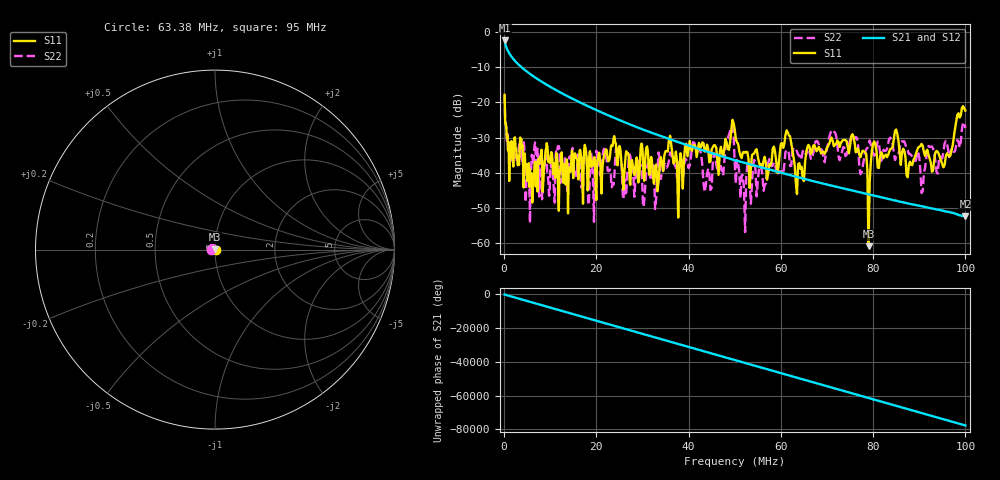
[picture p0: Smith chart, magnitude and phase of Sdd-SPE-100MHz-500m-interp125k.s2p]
!Keysight Technologies PLTS 2019, Build 20190114.1
!FILE: C:\Users\fxb06141\Documents\BUREAU - 2022\IEEE802.3\IEEE802.3dg\Cable modeling\125kHz Interpolation\SPE-100MHz-500m-interp125k.s4p
!$DUT_CFG_DESC: Default 4-Port Configuration
!$NUMBER_PORTS: 4
!$DIFF_PORT_MAP: 1|2P|2|2P|0|UC|0|UC|
!$PORT_MAP: 1|1|<<<<<<|2|2|>>>>>>|3|3|<<<<<<|4|4|>>>>>>|
!Date: Tuesday, March 05, 2024, 10:46:46
!S2P File: Measurements: SDD11,SDD12,SDD21,SDD22:
# MHz S  RI  R 50
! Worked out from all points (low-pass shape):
!   800 points, 125 kHz to 100 MHz, reference 50 ohm
!   highest |S21| = -2.50 dB at 125 kHz (marker M1); lowest = -52.3 dB at 100 MHz (marker M2)
!   |S21| within 3 dB of the highest: start of sweep to 858.2 kHz
!   lowest |S11| = -60.8 dB at 79 MHz (marker M3), VSWR 1.00, Z = 50 + j0.0913 ohm
!   |S11| at or under -10 dB: start of sweep to end of sweep
!   |S22| runs from -56.8 to -18.1 dB; largest |S21 - S12| = 0
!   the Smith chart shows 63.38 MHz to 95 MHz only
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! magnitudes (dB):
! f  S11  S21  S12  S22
! 125 kHz  -17.9  -2.5  -2.5  -18.1
! 1.5 MHz  -32.7  -6.9  -6.9  -31.2
! 5.125 MHz  -37.6  -11.5  -11.5  -40.4
! 6.375 MHz  -41.6  -12.7  -12.7  -37.5
! 16.88 MHz  -38.5  -20.3  -20.3  -43.7
! 23.75 MHz  -30.3  -24.4  -24.4  -43.3
! 33.5 MHz  -42.5  -29.4  -29.4  -34.2
! 41.5 MHz  -32.5  -32.9  -32.9  -32.3
! 43.62 MHz  -33.8  -33.9  -33.9  -44.5
! 49.25 MHz  -27.9  -36.2  -36.2  -27.1
! 50.12 MHz  -29.1  -36.5  -36.5  -40.1
! 51.88 MHz  -34.2  -37.1  -37.1  -42.5
! 63.62 MHz  -41.8  -41.2  -41.2  -34.4
! 66.75 MHz  -33.9  -42.3  -42.3  -36.2
! 75.62 MHz  -29.4  -45.1  -45.1  -30.4
! 77.5 MHz  -34.5  -45.6  -45.6  -39.8
! 79 MHz  -60.8  -46.1  -46.1  -31.8
! 80.12 MHz  -31.4  -46.4  -46.4  -34.8
! 83.38 MHz  -34.4  -47.4  -47.4  -31.0
! 90.75 MHz  -32.3  -49.6  -49.6  -45.2
! 95.25 MHz  -38.5  -50.8  -50.8  -33.9
! 100 MHz  -22.4  -52.3  -52.3  -27.3
